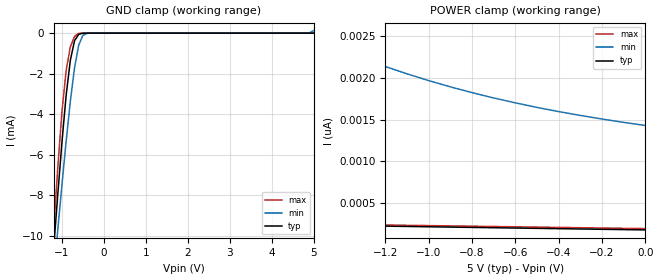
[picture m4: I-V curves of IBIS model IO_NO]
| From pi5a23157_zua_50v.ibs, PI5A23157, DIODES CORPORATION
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[Model]   IO_NO
Model_type   Terminator
C_comp   2.888pF   2.851pF   2.948pF
[Voltage Range]   5   4.5   5.5
[Temperature Range]   25   -40   125
[GND Clamp Reference]   0   0   0
[POWER Clamp Reference]   5   4.5   5.5
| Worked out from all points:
|   GND clamp passes 1 mA (typ) near -0.76 V on its own axis
[GND_Clamp]
-5V       -8.922A    -8.398A    -9.402A
-1.2V     -10.73mA   -12.06mA   -9.815mA
-1.1V     -8.002mA   -9.748mA   -6.689mA
-1V       -5.402mA   -7.504mA   -3.897mA
-900mV    -3.084mA   -5.355mA   -1.856mA
-800mV    -1.348mA   -3.375mA   -678.2uA
-700mV    -375.7uA   -1.713mA   -162uA
-600mV    -59.31uA   -592.2uA   -14.43uA
-500mV    -5.325uA   -108.5uA   -563.8nA
-400mV    -316.6nA   -10.9uA    -13.88nA
4.8V      508pA      2.336uA    422.7pA
5V        766.6pA    130.5uA    480.3pA
[Power_Clamp]
-5V       411.5pA    17.8nA     378.1pA
-3.5V     326.4pA    7.514nA    324pA
-1.6V     243.4pA    2.565nA    255.6pA
-1.4V     235.5pA    2.333nA    248.4pA
-1.3V     231.6pA    2.23nA     244.8pA
-1.2V     227.7pA    2.135nA    241.2pA
-1.1V     223.9pA    2.048nA    237.6pA
-900mV    216.2pA    1.892nA    230.4pA
-700mV    208.6pA    1.759nA    223.2pA
-500mV    201.1pA    1.646nA    216pA
-300mV    193.6pA    1.55nA     208.8pA
0V        182.5pA    1.43nA     198pA
